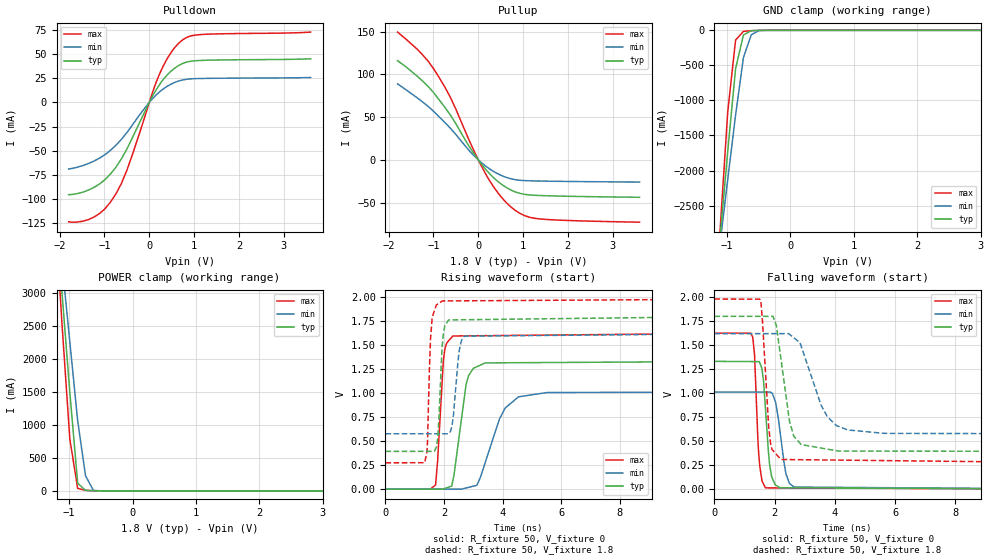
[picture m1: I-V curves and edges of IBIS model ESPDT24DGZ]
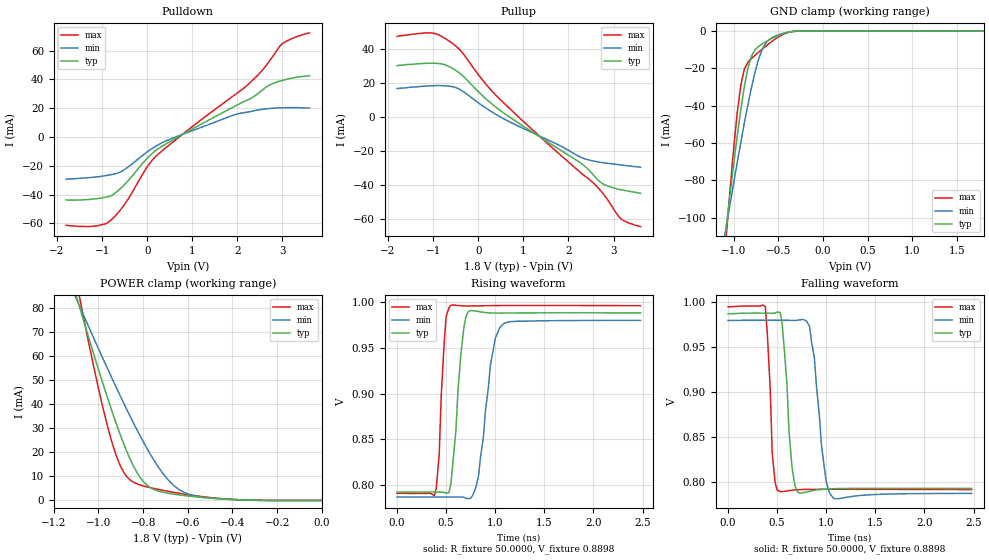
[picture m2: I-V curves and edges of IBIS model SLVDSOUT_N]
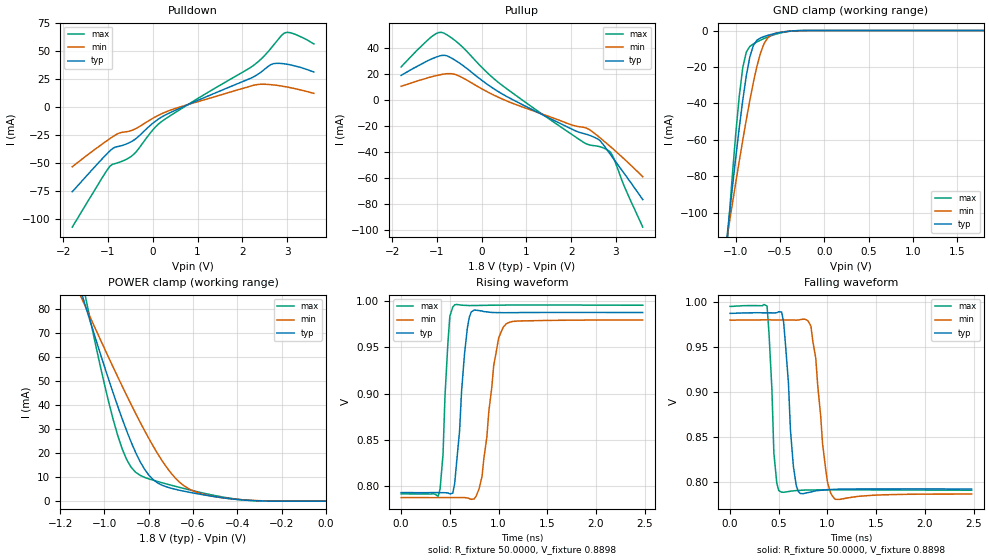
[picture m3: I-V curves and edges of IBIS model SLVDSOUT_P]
|   IBIS model for DLPC347x DMD CONTROLLER
[IBIS Ver]   4.1
[File name]   dlpc347x_v6.ibs
[File Rev]   1.0
[Date]   July 25, 2018
[Source]   Sigrity SpeedPKG Suite XtractIM 4.0.5.11011
[Notes]   One-Section RLC
[Disclaimer] Property of Texas Instruments Incorporated.  Unauthorized
   reproduction and/or distribution is strictly prohibited.
   This product is protected under copyright law.
   Created  2013, (C) Copyright  2013, Texas Instruments
   Incorporated, All Rights Reserved
   UNLESS THERE IS A SIGNED, WRITTEN AGREEMENT TO THE
   CONTRARY, TEXAS INSTRUMENTS (TI) IS PROVIDING THE IBIS
   MODELS  AND WITHOUT ANY WARRANTY, EXPRESSED OR
   IMPLIED.  TI assumes no liability for:
   1) the accuracy of the IBIS models provided to your
   company;
   2) the proper functioning of these IBIS Models in your
   design or for any resulting applications; or
   3) infringement of patents, copyrights or intellectual
   property rights resulting from your use of these IBIS
   models.
   TI provides IBIS Models as a service to our customers.
   You and your company shall not distribute, sell or give
   these models to anyone else without prior written
   permission from TI.
   TI reserves the right to make changes to our products or
   to discontinue any semiconductor product or service
   without notice, and advises our customers to obtain the
   latest version of relevant information to verify, before
   placing orders, that the information being relied on is
   current.
   Please be aware that your receipt and use of the IBIS
   information provided shall serve as acceptance of these
   terms and conditions.  If you do not accept these terms,
   you should return or destroy the IBIS models and any
   other accompanying information immediately.
|   Component DLPC347x
[Component] dlpc347x
[Manufacturer]  Texas Instruments
[Package]
|   typ   min   max
R_pkg   0.37693   0.031209   0.65717
L_pkg   3.735e-9   3.439e-10   6.55e-9
C_pkg   4.992e-13   2.684e-13   7.532e-12
[Pin]   Signal_name   model_name   R_pin   L_pin   C_pin
A12   CMP_OUT   PDISDGZ   0.44609   3.569e-9   3.596e-13
A15   CMP_PWM   PDB08DGZ_33   0.56775   5.309e-9   4.639e-13
P2   DATAEN_CMD   PDB08DGZ_33   0.50857   4.623e-9   4.445e-13
B1   DMD_DEN_ARSTZ   PDT04DGZ   0.64414   5.609e-9   5.102e-13
B7   DMD_HS_CLK_N   SLVDSOUT_N   0.38194   2.786e-9   3.53e-13
A7   DMD_HS_CLK_P   SLVDSOUT_P   0.3774   3.102e-9   3.242e-13
B11   DMD_HS_WDATA_A_N   SLVDSOUT_N   0.41554   3.461e-9   4.002e-13
A11   DMD_HS_WDATA_A_P   SLVDSOUT_P   0.45736   3.79e-9   3.944e-13
B10   DMD_HS_WDATA_B_N   SLVDSOUT_N   0.40053   3.367e-9   3.772e-13
A10   DMD_HS_WDATA_B_P   SLVDSOUT_P   0.43275   3.703e-9   3.683e-13
B9   DMD_HS_WDATA_C_N   SLVDSOUT_N   0.36884   2.966e-9   3.572e-13
A9   DMD_HS_WDATA_C_P   SLVDSOUT_P   0.39137   3.312e-9   3.313e-13
B8   DMD_HS_WDATA_D_N   SLVDSOUT_N   0.34855   2.803e-9   3.147e-13
A8   DMD_HS_WDATA_D_P   SLVDSOUT_P   0.37144   3.193e-9   3.021e-13
B6   DMD_HS_WDATA_E_N   SLVDSOUT_N   0.38571   2.995e-9   3.638e-13
A6   DMD_HS_WDATA_E_P   SLVDSOUT_P   0.39677   3.118e-9   3.299e-13
B5   DMD_HS_WDATA_F_N   SLVDSOUT_N   0.41659   3.456e-9   3.721e-13
A5   DMD_HS_WDATA_F_P   SLVDSOUT_P   0.41083   3.476e-9   3.499e-13
B4   DMD_HS_WDATA_G_N   SLVDSOUT_N   0.44793   3.772e-9   3.905e-13
A4   DMD_HS_WDATA_G_P   SLVDSOUT_P   0.44956   3.83e-9   3.706e-13
B3   DMD_HS_WDATA_H_N   SLVDSOUT_N   0.48652   4.243e-9   4.433e-13
A3   DMD_HS_WDATA_H_P   SLVDSOUT_P   0.47895   4.265e-9   3.91e-13
A1   DMD_LS_CLK   ESPDT24DGZ   0.54988   4.908e-9   4.467e-13
B2   DMD_LS_RDATA   PDIDGZ   0.46126   3.986e-9   4.103e-13
A2   DMD_LS_WDATA   ESPDT24DGZ   0.53434   4.65e-9   4.445e-13
C14   GPIO_00   PDB08SDGZ   0.46096   3.937e-9   3.99e-13
C15   GPIO_01   PDB08SDGZ   0.51963   4.535e-9   3.998e-13
D14   GPIO_02   PDB08SDGZ   0.42622   3.751e-9   3.855e-13
D15   GPIO_03   PDB08SDGZ   0.48192   4.333e-9   3.808e-13
E14   GPIO_04   PDB08SDGZ   0.3885   3.443e-9   3.519e-13
E15   GPIO_05   PDB08SDGZ   0.45545   4.095e-9   3.445e-13
F14   GPIO_06   PDB08SDGZ   0.36884   3.188e-9   3.33e-13
F15   GPIO_07   PDB08SDGZ   0.43264   3.826e-9   3.259e-13
G14   GPIO_08   PDB08SDGZ   0.33682   2.795e-9   3.077e-13
G15   GPIO_09   PDB08SDGZ   0.42938   3.836e-9   3.395e-13
H14   GPIO_10   PDB08SDGZ   0.36129   3.052e-9   3.405e-13
H15   GPIO_11   PDB08SDGZ   0.42185   3.591e-9   3.35e-13
J14   GPIO_12   PDB08SDGZ   0.39927   3.25e-9   3.569e-13
J15   GPIO_13   PDB08SDGZ   0.4411   3.695e-9   3.534e-13
K14   GPIO_14   PDB08SDGZ   0.53886   4.881e-9   4.101e-13
K15   GPIO_15   PDB08SDGZ   0.45165   4.097e-9   3.451e-13
L14   GPIO_16   PDB08SDGZ   0.45901   4.075e-9   3.419e-13
L15   GPIO_17   PDB08SDGZ   0.45656   4.189e-9   3.503e-13
M14   GPIO_18   PDB08SDGZ   0.58635   5.319e-9   3.902e-13
M15   GPIO_19   PDB08SDGZ   0.49904   4.591e-9   3.768e-13
N8   HOST_IRQ   PDB08DGZ_33   0.3009   2.663e-9   2.959e-13
N5   HSYNC_CS   PDB08DGZ_33   0.33725   2.925e-9   3.568e-13
C10   HWTEST_EN   PDIDGZ   0.30242   2.424e-9   4.426e-13
N10   IIC0_SCL   eSI2CSFTPZ   0.35938   2.815e-9   3.681e-13
N9   IIC0_SDA   eSI2CSFTPZ   0.31231   2.732e-9   3.229e-13
B15   LED_SEL_0   PDB08DGZ_33   0.53703   4.854e-9   4.213e-13
B14   LED_SEL_1   PDB08DGZ_33   0.49156   4.544e-9   4.234e-13
C13   PARKZ   PDISDGZ   0.69615   6.596e-9   4.641e-13
P3   PCLK   PDB08DGZ_33   0.43133   3.924e-9   3.611e-13
K2   PDATA_0   PDB08DGZ_33   0.39647   3.263e-9   3.689e-13
K1   PDATA_1   PDB08DGZ_33   0.40977   3.366e-9   3.288e-13
L2   PDATA_2   PDB08DGZ_33   0.41762   3.416e-9   3.533e-13
L1   PDATA_3   PDB08DGZ_33   0.43024   3.606e-9   3.284e-13
M2   PDATA_4   PDB08DGZ_33   0.43595   3.692e-9   3.421e-13
M1   PDATA_5   PDB08DGZ_33   0.4628   3.905e-9   3.326e-13
N2   PDATA_6   PDB08DGZ_33   0.48207   4.046e-9   3.843e-13
N1   PDATA_7   PDB08DGZ_33   0.51206   4.346e-9   3.895e-13
R1   PDATA_8   PDB08DGZ_33   0.53734   4.986e-9   4.232e-13
R2   PDATA_9   PDB08DGZ_33   0.48804   4.526e-9   3.676e-13
R3   PDATA_10   PDB08DGZ_33   0.48003   4.451e-9   3.765e-13
P4   PDATA_11   PDB08DGZ_33   0.40478   3.623e-9   3.505e-13
R4   PDATA_12   PDB08DGZ_33   0.45372   4.177e-9   3.44e-13
P5   PDATA_13   PDB08DGZ_33   0.37448   3.347e-9   3.28e-13
R5   PDATA_14   PDB08DGZ_33   0.42246   3.941e-9   3.173e-13
P6   PDATA_15   PDB08DGZ_33   0.35345   2.997e-9   3.262e-13
R6   PDATA_16   PDB08DGZ_33   0.41986   3.867e-9   3.357e-13
P7   PDATA_17   PDB08DGZ_33   0.35483   2.962e-9   3.448e-13
R7   PDATA_18   PDB08DGZ_33   0.39713   3.67e-9   3.002e-13
P8   PDATA_19   PDB08DGZ_33   0.33483   2.877e-9   3.123e-13
R8   PDATA_20   PDB08DGZ_33   0.39305   3.487e-9   3.016e-13
P9   PDATA_21   PDB08DGZ_33   0.35662   3.287e-9   3.03e-13
R9   PDATA_22   PDB08DGZ_33   0.41718   3.597e-9   3.345e-13
P10   PDATA_23   PDB08DGZ_33   0.39771   3.349e-9   3.44e-13
N4   PDM_CVS_TE   PDB08DGZ_33   0.38977   3.488e-9   3.827e-13
H1   PLL_REFCLK_I   no_model   0.36383   3.263e-9   3.169e-13
J1   PLL_REFCLK_O   no_model   0.39133   3.613e-9   3.366e-13
C11   RESETZ   PDISDGZ   0.61208   5.376e-9   4.319e-13
N6   3DR   PDB08DGZ_33   0.32215   2.848e-9   3.159e-13
A13   SPI0_CLK   PDB08DGZ_25   0.50095   4.2e-9   3.54e-13
A14   SPI0_CSZ0   PDUW08DGZ   0.4888   4.168e-9   3.348e-13
C12   SPI0_CSZ1   PDUW08DGZ   0.36968   2.702e-9   3.51e-13
B12   SPI0_DIN   PDIDGZ_25   0.37381   3.331e-9   3.799e-13
B13   SPI0_DOUT   PDB08DGZ_25   0.45044   3.887e-9   3.758e-13
R12   TSTPT_0   PDDW08DGZ   0.48168   4.361e-9   3.67e-13
R13   TSTPT_1   PDDW08DGZ   0.6056   4.896e-9   5.182e-13
R14   TSTPT_2   PDDW08DGZ   0.54873   5.108e-9   4.539e-13
R15   TSTPT_3   PDDW08DGZ   0.60219   5.633e-9   4.746e-13
P14   TSTPT_4   PDDW08DGZ   0.53834   4.905e-9   4.562e-13
P15   TSTPT_5   PDDW08DGZ   0.59898   5.234e-9   4.41e-13
N14   TSTPT_6   PDDW08DGZ   0.53088   4.748e-9   3.766e-13
N15   TSTPT_7   PDDW08DGZ   0.5036   4.297e-9   3.833e-13
P1   VSYNC_WE   PDB08DGZ_33   0.57379   5.176e-9   4.379e-13
|   MODEL no_model
[Model]   no_model
Model_type   Input
Vinl  = 0.6V
Vinh  = 1.2V
|   typ   min   max
C_comp   1pf   1pf   1pf
[Temperature Range]   25   100   -40
[Voltage Range]   1.8   1.7   1.9
|End [Model]  no_model
|   MODEL no_model_Arasan
[Model]   no_model_Arasan
Model_type   Input
Vinl  = 0.6V
Vinh  = 1.2V
|   typ   min   max
C_comp   1pf   1pf   1pf
[Temperature Range]   25   100   -40
[Voltage Range]   1.8   1.7   1.9
|End [Model]  no_model_Arasan
| Models and submodels in the file (17): no_model (Input), no_model_Arasan (Input), ESPDT24DGZ (3-state), SLVDSOUT_N (3-state), SLVDSOUT_P (3-state), eSI2CSFTPZ (I/O_open_drain), PDISDGZ (Input), PDT04DGZ (3-state), PDIDGZ (Input), PDB08SDGZ (I/O), PDUDGZ (Input), PDT08DGZ (3-state), PDUW08DGZ (I/O), PDDW08DGZ (I/O), PDB08DGZ_33 (I/O), PDB08DGZ_25 (I/O), PDIDGZ_25 (Input)
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[Model] ESPDT24DGZ
Model_type 3-state
Polarity  Non-Inverting
Enable   Active-Low
Vmeas =  0.9
| Capacitance   typ   min   max
C_comp   1.49607136358e-12   1.64847775117e-12   1.35395807733e-12
| Variables   typ   min   max
[GND Clamp Reference]   0   0   0
[POWER Clamp Reference]   1.8   1.62   1.98
[Pulldown Reference]   0   0   0
[Pullup Reference]   1.8   1.62   1.98
[Temperature Range]   25   105   -40
[Voltage Range]   1.8   1.62   1.98
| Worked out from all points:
|   slope of the pulldown table from 0 to 0.27 V, typ, clamps not added: 12.8 ohm
|   slope of the pullup table from 0 to 0.27 V, typ, clamps not added: 15.8 ohm
|   GND clamp passes 1 mA (typ) near -0.50 V on its own axis
|   POWER clamp passes 1 mA (typ) near -0.52 V on its own axis
|   falling waveform, R_fixture 50, V_fixture 0: 20-80 % time 184ps typ, 268ps min, 138ps max; typ from 1.33 V to 0 V
|   falling waveform, R_fixture 50, V_fixture 1.8: 20-80 % time 385ps typ, 732ps min, 196ps max; typ from 1.8 V to 0.394 V
|   rising waveform, R_fixture 50, V_fixture 0: 20-80 % time 348ps typ, 699ps min, 183ps max; typ from 0 V to 1.33 V
|   rising waveform, R_fixture 50, V_fixture 1.8: 20-80 % time 133ps typ, 182ps min, 111ps max; typ from 0.394 V to 1.8 V
[GND Clamp]
| Voltage   I(typ)   I(min)   I(max)
-1.8V     -10.22A    -8.383A    -13.02A
-1.114V   -2.984A    -3.062A    -2.89A
-990mV    -1.723A    -2.125A    -1.159A
-866.2mV  -546mA     -1.208A    -139.3mA
-742.5mV  -66.28mA   -388.2mA   -14.78mA
-618.8mV  -5.042mA   -63.31mA   -5.078mA
-495mV    -895.8uA   -3.147mA   -786.1uA
3.6V      0A         0A         0A
[POWER Clamp]
| Voltage   I(typ)   I(min)   I(max)
-1.8V     11.44A     10.1A      13.31A
-1.238V   4.531A     4.656A     4.477A
-1.114V   3.013A     3.459A     2.536A
-990mV    1.496A     2.263A     788.8mA
-866.2mV  118.8mA    1.065A     38.51mA
-742.5mV  8.288mA    231.4mA    9.621mA
-618.8mV  2.794mA    8.479mA    3.645mA
3.6V      0A         0A         0A
[Pulldown]
| Voltage   I(typ)   I(min)   I(max)
-1.8V     -95.62mA   -69.03mA   -123.8mA
-1.485V   -93.07mA   -65.52mA   -123.2mA
-1.238V   -88.22mA   -60.89mA   -119mA
-990mV    -80.12mA   -54.19mA   -110.3mA
-742.5mV  -67.02mA   -44.34mA   -94.68mA
-495mV    -47.89mA   -30.98mA   -69.69mA
28.13mV   2.616mA    1.543mA    4.178mA
225mV     18.19mA    10.72mA    28.98mA
478.1mV   32.04mA    18.75mA    51.14mA
731.2mV   40.03mA    23.12mA    64.31mA
1.181V    43.57mA    24.82mA    70.42mA
3.6V      45.18mA    25.8mA     72.88mA
[Pullup]
| Voltage   I(typ)   I(min)   I(max)
-1.8V     116mA      88.86mA    149.5mA
-1.361V   97.9mA     72.54mA    129.4mA
-1.114V   85.64mA    62.37mA    115.2mA
-990mV    78.31mA    56.45mA    106.1mA
-618.8mV  52.22mA    36.81mA    72.79mA
-123.7mV  9.369mA    6.374mA    13.77mA
196.9mV   -12.93mA   -8.523mA   -19.38mA
478.1mV   -27mA      -17.39mA   -41.24mA
787.5mV   -36.71mA   -22.84mA   -57.64mA
1.041V    -40.42mA   -24.33mA   -65.39mA
1.35V     -41.7mA    -24.8mA    -69.04mA
3.6V      -43.86mA   -26.04mA   -73mA
[Ramp]
dV/dt_r   0.798662/0.348448n  0.607012/0.698993n  0.975045/0.182835n
dV/dt_f   0.843734/0.385318n  0.625915/0.732458n  1.0233/0.196216n
R_load = 50
[Falling Waveform]
R_fixture = 50
V_fixture = 0
V_fixture_min = 0
V_fixture_max = 0
| Time   V(typ)   V(min)   V(max)
0s        1.331V     1.012V     1.625V
1.272ns   1.329V     1.012V     1.584V
1.332ns   1.329V     1.012V     1.399V
1.491ns   1.328V     1.012V     294.8mV
1.631ns   1.129V     1.012V     53.41mV
1.696ns   831.2mV    1.012V     13.25mV
1.901ns   127.5mV    1.003V     13mV
2.375ns   15.16mV    160.7mV    12.41mV
2.647ns   14.75mV    22.18mV    12.08mV
12.46ns   5.021nV    31.8nV     363.3pV
[Falling Waveform]
R_fixture = 50
V_fixture = 1.8
V_fixture_min = 1.62
V_fixture_max = 1.98
| Time   V(typ)   V(min)   V(max)
0s        1.8V       1.62V      1.98V
1.539ns   1.8V       1.62V      1.967V
1.87ns    1.8V       1.62V      464.9mV
2.057ns   1.705V     1.62V      362.4mV
2.208ns   1.358V     1.62V      309.1mV
2.491ns   710.2mV    1.613V     308.2mV
2.882ns   464.1mV    1.487V     306.8mV
3.747ns   417.3mV    756mV      303.9mV
4.421ns   396.2mV    617.2mV    301.6mV
12.46ns   393.8mV    576.8mV    274.5mV
[Rising Waveform]
R_fixture = 50
V_fixture = 0
V_fixture_min = 0
V_fixture_max = 0
| Time   V(typ)   V(min)   V(max)
0s        1.042nV    33.56nV    374.9pV
1.709ns   1.042nV    33.56nV    42.51mV
1.975ns   3.663mV    33.56nV    1.343V
2.301ns   93.6mV     33.56nV    1.595V
2.748ns   1.087V     11.97mV    1.597V
3.12ns    1.276V     40.99mV    1.598V
3.404ns   1.315V     278.1mV    1.599V
3.886ns   1.316V     729mV      1.6V
4.541ns   1.317V     962mV      1.602V
12.46ns   1.331V     1.012V     1.625V
[Rising Waveform]
R_fixture = 50
V_fixture = 1.8
V_fixture_min = 1.62
V_fixture_max = 1.98
| Time   V(typ)   V(min)   V(max)
0s        393.8mV    576.8mV    274.5mV
1.337ns   393.8mV    576.8mV    275.6mV
1.433ns   393.8mV    576.8mV    487.6mV
1.501ns   393.8mV    576.8mV    1.269V
1.594ns   393.8mV    576.8mV    1.79V
1.782ns   530.3mV    576.8mV    1.928V
1.944ns   1.513V     576.8mV    1.96V
2.271ns   1.763V     665.2mV    1.961V
2.688ns   1.765V     1.593V     1.962V
12.46ns   1.8V       1.62V      1.98V
[Model] SLVDSOUT_N
Model_type 3-state
Polarity   Inverting
Enable   Active-Low
Vmeas =  0.9000V
Rref =   50.0000
Vref =   0.9000V
C_comp   2.1155pF   1.9207pF   2.4381pF
[Temperature Range]   25.0000   0.1250k   -40.0000
[Pullup Reference]   1.8000V   1.6200V   1.9800V
[Pulldown Reference]   0.0V   0.0V   0.0V
[POWER Clamp Reference]   1.8000V   1.6200V   1.9800V
[GND Clamp Reference]   0.0V   0.0V   0.0V
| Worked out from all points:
|   slope of the pulldown table from 0 to 0.27 V, typ, clamps not added: 37.5 ohm
|   slope of the pullup table from 0 to 0.27 V, typ, clamps not added: 41.3 ohm
|   GND clamp passes 1 mA (typ) near -0.42 V on its own axis
|   POWER clamp passes 1 mA (typ) near -0.50 V on its own axis
|   rising waveform, R_fixture 50.0000, V_fixture 0.8898: 20-80 % time 81.6ps typ, 124ps min, 51.5ps max; typ from 0.793 V to 0.988 V
|   falling waveform, R_fixture 50.0000, V_fixture 0.8898: 20-80 % time 67.5ps typ, 95.2ps min, 45ps max; typ from 0.987 V to 0.793 V
[Pulldown]
|Voltage   I(typ)   I(min)   I(max)
-1.8V     -43.7mA    -29.3mA    -61.3mA
-1.2V     -43.1mA    -28mA      -62mA
-840mV    -41.24mA   -26.36mA   -58.7mA
-540mV    -34.19mA   -23.36mA   -48.43mA
0V        -14.82mA   -10.37mA   -20.76mA
180mV     -9.621mA   -6.626mA   -13.74mA
600mV     -1.471mA   -349.2uA   -2.739mA
1.98V     21.96mA    15.78mA    30.15mA
2.52V     31.73mA    19.04mA    45.17mA
2.7V      35.86mA    19.71mA    52.24mA
3V        39.3mA     20.3mA     64.87mA
3.6V      42.5mA     20.1mA     72.3mA
[Pullup]
|Voltage   I(typ)   I(min)   I(max)
-1.8V     30.4mA     16.9mA     47.6mA
-1.02V    31.83mA    18.56mA    49.57mA
-780mV    31.23mA    18.56mA    47.14mA
-540mV    28.31mA    17.84mA    42.84mA
-360mV    24.89mA    15.64mA    38.31mA
60mV      13.63mA    7.445mA    23.15mA
420mV     5.387mA    1.304mA    12.21mA
2.28V     -27mA      -23.58mA   -32.76mA
2.58V     -34.73mA   -25.86mA   -39.31mA
2.76V     -39.03mA   -26.7mA    -44.62mA
3.18V     -42.7mA    -28.1mA    -60.1mA
3.6V      -44.7mA    -29.4mA    -64.3mA
[GND_clamp]
|Voltage   I(typ)   I(min)   I(max)
-1.8V     -422mA     -319.8mA   -581.8mA
-1.12V    -120.3mA   -115.5mA   -132.3mA
-1.08V    -103.6mA   -104mA     -108mA
-960mV    -56.13mA   -70.36mA   -43.62mA
-920mV    -41.99mA   -59.62mA   -28.87mA
-880mV    -29.52mA   -49.23mA   -20.31mA
-800mV    -13.27mA   -30.08mA   -14.64mA
-720mV    -8.152mA   -14.87mA   -11.26mA
-640mV    -5.72mA    -6.44mA    -8.062mA
-560mV    -3.686mA   -3.243mA   -5.122mA
-280mV    -46.98uA   -91.92uA   -30.72uA
1.8V      9.267nA    13.2uA     412pA
[POWER_clamp]
|Voltage   I(typ)   I(min)   I(max)
-1.8V     320.5mA    240.3mA    452mA
-1.1V     85.37mA    84.19mA    91.82mA
-1.08V    79.06mA    79.94mA    82.36mA
-1V       54.51mA    63.18mA    46.63mA
-940mV    37.27mA    50.96mA    24.31mA
-900mV    26.75mA    43.05mA    13.96mA
-860mV    17.55mA    35.39mA    8.647mA
-780mV    6.139mA    21.23mA    5.591mA
-700mV    3.195mA    9.886mA    4.017mA
-620mV    2.109mA    3.549mA    2.716mA
-440mV    594.6uA    619.7uA    724.9uA
0V        9.266nA    150.2nA    995.7pA
[Ramp]
| variable   typ   min   max
dV/dt_r 0.1953/0.0757n   0.1926/0.1181n   0.2046/0.0510n
dV/dt_f 0.1945/0.0618n   0.1925/0.0932n   0.2035/0.0450n
R_load = 50.0000
[Rising Waveform]
R_fixture= 50.0000
V_fixture= 0.8898
V_fixture_min= 0.8834
V_fixture_max= 0.8930
|time   V(typ)   V(min)   V(max)
0s        792.6mV    787.2mV    791.2mV
380ps     792.6mV    787.2mV    788.5mV
430ps     792.5mV    787.2mV    834mV
500ps     791.2mV    787.2mV    983.9mV
550ps     802.9mV    787.2mV    996.3mV
720ps     988.5mV    785.3mV    995.5mV
830ps     989.5mV    810mV      995.6mV
950ps     987.9mV    930.3mV    995.8mV
1.08ns    987.7mV    975.8mV    996mV
2.48ns    987.9mV    979.8mV    995.8mV
[Falling Waveform]
R_fixture= 50.0000
V_fixture= 0.8898
V_fixture_min= 0.8834
V_fixture_max= 0.8930
|time   V(typ)   V(min)   V(max)
0s        987.1mV    979.6mV    994.8mV
380ps     987.7mV    979.9mV    995.2mV
450ps     987.5mV    979.8mV    832.3mV
500ps     988.9mV    979.8mV    790.9mV
550ps     977.4mV    979.8mV    789mV
720ps     787.7mV    980.1mV    791.2mV
830ps     789.3mV    973mV      791.6mV
1ns       791.9mV    800.3mV    791.7mV
1.08ns    792.3mV    781.2mV    791.7mV
2.48ns    792.6mV    787.1mV    791.3mV
[Model]  SLVDSOUT_P
Model_type 3-state
Polarity   Non-Inverting
Enable   Active-Low
Vmeas =  0.9000V
Rref =   50.0000
Vref =   0.9000V
C_comp   2.1155pF   1.9207pF   2.4381pF
[Temperature Range]   25.0000   0.1250k   -40.0000
[Pullup Reference]   1.8000V   1.6200V   1.9800V
[Pulldown Reference]   0.0V   0.0V   0.0V
[POWER Clamp Reference]   1.8000V   1.6200V   1.9800V
[GND Clamp Reference]   0.0V   0.0V   0.0V
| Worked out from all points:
|   slope of the pulldown table from 0 to 0.27 V, typ, clamps not added: 37.5 ohm
|   slope of the pullup table from 0 to 0.27 V, typ, clamps not added: 41.3 ohm
|   GND clamp passes 1 mA (typ) near -0.49 V on its own axis
|   POWER clamp passes 1 mA (typ) near -0.43 V on its own axis
|   rising waveform, R_fixture 50.0000, V_fixture 0.8898: 20-80 % time 81.6ps typ, 124ps min, 51.5ps max; typ from 0.793 V to 0.988 V
|   falling waveform, R_fixture 50.0000, V_fixture 0.8898: 20-80 % time 67.5ps typ, 95.2ps min, 45ps max; typ from 0.987 V to 0.793 V
[Pulldown]
|Voltage   I(typ)   I(min)   I(max)
-1.8V     -75.9mA    -53.6mA    -107.5mA
-960mV    -39.5mA    -28.52mA   -53.23mA
-840mV    -36.05mA   -25.37mA   -50.76mA
-720mV    -35.05mA   -23.13mA   -49.2mA
-420mV    -29.76mA   -20.33mA   -42.29mA
0V        -14.82mA   -10.37mA   -20.76mA
180mV     -9.621mA   -6.626mA   -13.74mA
2.22V     25.99mA    18.75mA    35.96mA
2.64V     37.57mA    19.63mA    52.04mA
2.94V     38.26mA    18mA       65.71mA
3.12V     36.9mA     16.6mA     65.5mA
3.6V      31mA       11.9mA     56mA
[Pullup]
|Voltage   I(typ)   I(min)   I(max)
-1.8V     18.9mA     10.5mA     25.4mA
-1.02V    32.99mA    18.68mA    51.07mA
-900mV    34.23mA    19.58mA    52.1mA
-720mV    33.1mA     20.27mA    48.92mA
-480mV    28.03mA    18mA       42.43mA
300mV     7.947mA    3.225mA    15.55mA
960mV     -4.549mA   -6.075mA   -1.394mA
2.28V     -25.94mA   -21.13mA   -32.75mA
2.58V     -29.84mA   -27.37mA   -35.62mA
2.88V     -42.2mA    -36.1mA    -40.29mA
3.18V     -56.5mA    -45.4mA    -66.1mA
3.6V      -76.9mA    -59.3mA    -98.1mA
[GND_clamp]
|Voltage   I(typ)   I(min)   I(max)
-1.8V     -454.2mA   -344.1mA   -628mA
-1.12V    -123.5mA   -120.9mA   -133.4mA
-1.08V    -105.3mA   -108.3mA   -106.7mA
-1V       -70.12mA   -83.81mA   -57.26mA
-920mV    -38.27mA   -60.24mA   -20.42mA
-880mV    -24.85mA   -49.01mA   -11.85mA
-840mV    -14.47mA   -38.33mA   -8.73mA
-800mV    -8.164mA   -28.42mA   -7.318mA
-720mV    -4.06mA    -12.38mA   -5.293mA
-640mV    -2.676mA   -4.114mA   -3.594mA
-440mV    -627uA     -587.5uA   -769.6uA
1.8V      9.267nA    13.84uA    416.3pA
[POWER_clamp]
|Voltage   I(typ)   I(min)   I(max)
-1.8V     309mA      233.9mA    429.8mA
-1.1V     85.42mA    83.71mA    91.36mA
-1.08V    79.4mA     79.61mA    82.42mA
-1V       55.93mA    63.44mA    48.55mA
-940mV    39.4mA     51.64mA    27.26mA
-900mV    29.27mA    44mA       17.32mA
-860mV    20.37mA    36.59mA    12.06mA
-760mV    7.576mA    19.75mA    8.157mA
-680mV    4.919mA    9.584mA    6.164mA
-600mV    3.398mA    4.27mA     4.322mA
-360mV    364.7uA    456.7uA    413.3uA
0V        9.266nA    150.2nA    999.8pA
[Ramp]
| variable   typ   min   max
dV/dt_r 0.1953/0.0757n   0.1926/0.1181n   0.2046/0.0510n
dV/dt_f 0.1945/0.0618n   0.1925/0.0932n   0.2035/0.0450n
R_load = 50.0000
[Rising Waveform]
R_fixture= 50.0000
V_fixture= 0.8898
V_fixture_min= 0.8834
V_fixture_max= 0.8930
|time   V(typ)   V(min)   V(max)
0s        792.6mV    787.2mV    791.2mV
380ps     792.6mV    787.2mV    788.5mV
430ps     792.5mV    787.2mV    834mV
500ps     791.2mV    787.2mV    983.9mV
550ps     802.9mV    787.2mV    996.3mV
720ps     988.5mV    785.3mV    995.5mV
830ps     989.5mV    810mV      995.6mV
950ps     987.9mV    930.3mV    995.8mV
1.08ns    987.7mV    975.8mV    996mV
2.48ns    987.9mV    979.8mV    995.8mV
[Falling Waveform]
R_fixture= 50.0000
V_fixture= 0.8898
V_fixture_min= 0.8834
V_fixture_max= 0.8930
|time   V(typ)   V(min)   V(max)
0s        987.1mV    979.6mV    994.8mV
380ps     987.7mV    979.9mV    995.2mV
450ps     987.5mV    979.8mV    832.3mV
500ps     988.9mV    979.8mV    790.9mV
550ps     977.4mV    979.8mV    789mV
720ps     787.7mV    980.1mV    791.2mV
830ps     789.3mV    973mV      791.6mV
1ns       791.9mV    800.3mV    791.7mV
1.08ns    792.3mV    781.2mV    791.7mV
2.48ns    792.6mV    787.1mV    791.3mV
